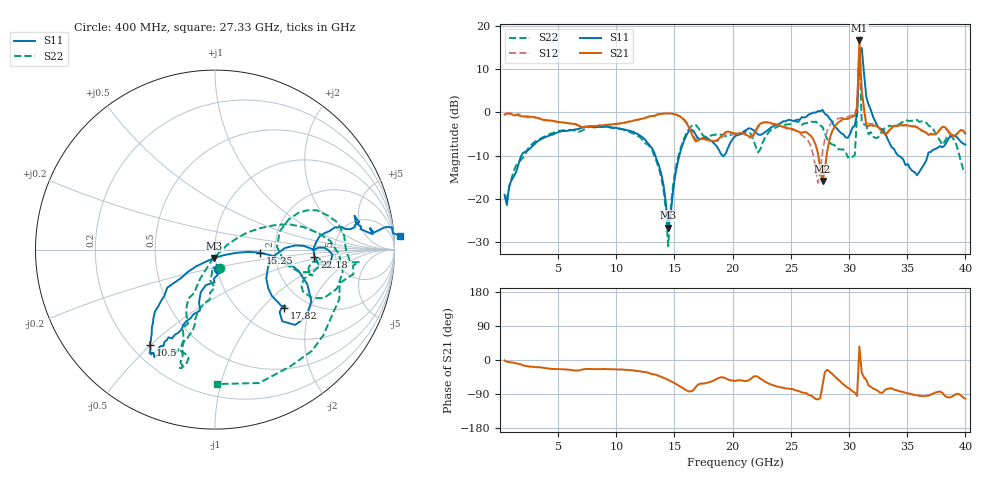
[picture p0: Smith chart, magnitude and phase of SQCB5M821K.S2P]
! Network Analyzer HP8722ES.07.66: Jul 25, 2000 Serial No. US39175408
! 27 Oct 2004  14:52:11
! Frequency  S11  S21  S12  S22
# HZ  S  DB R  50
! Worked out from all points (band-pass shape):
!   201 points, 400 MHz to 40 GHz, reference 50 ohm
!   highest |S21| = 16.65 dB at 30.89 GHz (marker M1); lowest = -15.9 dB at 27.72 GHz (marker M2)
!   |S21| within 3 dB of the highest: 30.85344 GHz to 30.94298 GHz (89.54 MHz wide, 0.29 % of centre)
!   lowest |S11| = -26.6 dB at 14.46 GHz (marker M3), VSWR 1.10, Z = 49.4 - j4.59 ohm
!   |S11| at or under -10 dB: start of sweep to 1.843 GHz; 13.35 GHz to 15.42 GHz (2.067 GHz wide, 14.4 % of centre); 34.24 GHz to 36.75 GHz (2.516 GHz wide, 7.09 % of centre)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
!   |S22| runs from -31.0 to 14.7 dB; largest |S21 - S12| = 2.3
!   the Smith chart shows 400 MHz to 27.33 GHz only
!   S11 on the Smith chart (normalised r, x): 400 MHz: 1.01, -0.22; 10.5 GHz: 0.27, -0.50; 15.25 GHz: 1.67, -0.06; 17.82 GHz: 1.55, -1.34; 22.18 GHz: 3.45, -0.39; 27.33 GHz: -10, +22
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4e8  -19.08 -82.3  -0.55 -1.3  -0.53 -0.5  -19.66 -75.3
7.132e9  -3.47 -118.6  -3.42 -24.9  -3.52 -26.1  -4.12 -103.7
1.0498e10  -3.84 -124.2  -2.46 -25.1  -2.48 -25.7  -3.94 -106.9
1.3666e10  -12.33 -140.0  -0.45 -42.1  -0.38 -42.3  -12.99 -116.5
1.4458e10  -26.64 -94.8  -0.25 -52.5  -0.16 -52.6  -30.96 -49.1
1.525e10  -11.93 -3.9  -0.66 -65.3  -0.57 -65.4  -11.06 25.3
1.7824e10  -5.98 -40.1  -6.35 -60.1  -6.25 -63.4  -5.67 -19.0
2.02e10  -5.52 0.9  -4.85 -55.1  -5.07 -55.4  -4.95 -6.8
2.218e10  -5.10 -4.0  -3.18 -44.5  -3.45 -44.0  -9.24 2.7
2.6932e10  -0.05 7.1  -6.28 -97.8  -9.96 -101.3  -2.22 -57.2
2.7328e10  0.29 4.3  -9.43 -104.1  -16.38 -66.7  -2.51 -89.3
2.7724e10  0.57 -2.6  -15.85 -66.7  -8.98 -14.2  -3.34 -130.6
2.8714e10  -3.15 -16.7  -3.60 -41.5  -1.86 -50.0  -7.49 120.8
2.9902e10  -5.87 5.4  -1.51 -73.5  -1.01 -77.6  -10.46 77.4
3.0694e10  -0.22 20.5  1.25 -94.7  1.46 -96.3  -0.51 127.6
3.0892e10  14.52 116.6  16.65 35.5  13.96 21.5  14.71 -70.2
3.109e10  14.91 0.2  5.00 -32.9  4.94 -35.8  -2.28 -67.2
3.1288e10  8.99 -35.1  0.81 -46.1  0.94 -48.1  -2.75 -45.2
3.1684e10  1.78 -55.8  -3.15 -67.5  -2.59 -69.9  -5.07 -45.2
3.3466e10  -7.00 -84.6  -4.10 -75.0  -4.04 -76.7  -3.03 -140.8
3.703e10  -9.13 97.6  -5.01 -91.2  -4.88 -91.9  -3.34 127.8
4e10  -7.45 57.5  -4.87 -102.1  -5.01 -103.0  -13.94 59.6
